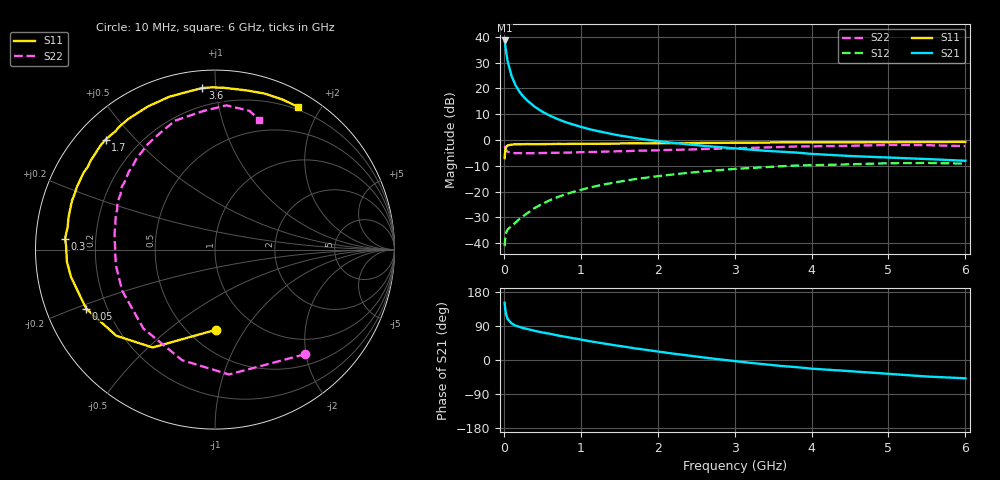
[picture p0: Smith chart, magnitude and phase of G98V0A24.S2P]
! SIEMENS Small Signal Semiconductors
! BFG235
! Si NPN RF Bipolar Junction Transistor in SOT223
! VCE = 8 V  IC = 240 mA
! Common Emitter S-Parameters:  July  1994
# GHz  S  MA  R  50
!  f  S11  S21  S12  S22
! GHz  MAG  ANG  MAG  ANG  MAG  ANG  MAG  ANG
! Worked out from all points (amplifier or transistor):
!   40 points, 10 MHz to 6 GHz, reference 50 ohm
!   highest |S21| = 38.6 dB at 10 MHz (marker M1)
!   |S21| within 3 dB of that: start of sweep to 23.42 MHz
!   unconditionally stable (mu >= 1): 421.9 MHz to 1.53 GHz
!   at 200 MHz: K = 0.83, MSG = 24.8 dB, |S12| = -30.7 dB
!   at 1.5 GHz: K = 1.00, MAG = 8.5 dB, |S12| = -16.1 dB
!   at 6 GHz: K = 0.89, MSG = 0.5 dB, |S12| = -9.1 dB
!   S11 on the Smith chart (normalised r, x): 10 MHz: 0.67, -0.75; 50 MHz: 0.12, -0.21; 300 MHz: 0.09, +0.04; 1.7 GHz: 0.09, +0.41; 3.6 GHz: 0.09, +0.92; 6 GHz: 0.17, +1.72
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0.01  0.4474 -89.6  85.11 150.8  0.0088 59.2  0.7689 -49.3
0.02  0.6466 -122.5  65.85 131.4  0.0139 47.0  0.7002 -83.6
0.03  0.73 -138.9  50.78 119.8  0.0163 39.9  0.6427 -106.6
0.05  0.7894 -155.4  33.39 107.9  0.0186 33.3  0.5937 -132.2
0.1  0.817 -169.3  17.51 96.7  0.0215 38.7  0.5657 -155.9
0.15  0.8279 -175.5  11.74 90.9  0.0251 45.2  0.5571 -165.9
0.2  0.8281 -179.0  8.786 87.5  0.0293 50.1  0.5594 -171.0
0.25  0.8306 178.1  7.073 84.3  0.0335 53.8  0.5563 -174.6
0.3  0.8377 175.9  5.906 81.9  0.0379 56.6  0.5567 -177.8
0.4  0.8306 171.3  4.44 77.0  0.0482 59.5  0.5566 178.2
0.5  0.8353 167.7  3.546 72.7  0.058 61.1  0.5615 174.9
0.6  0.8375 164.7  2.961 69.1  0.0684 61.0  0.5654 171.8
0.8  0.8413 158.3  2.234 61.2  0.0889 59.9  0.5699 166.5
1.1  0.8485 149.3  1.643 50.1  0.1185 56.0  0.5865 159.7
1.4  0.8536 142.2  1.314 40.2  0.1466 51.1  0.6032 153.6
1.7  0.8639 134.8  1.102 30.8  0.1747 45.8  0.6204 148.0
2.2  0.8735 123.7  0.883 16.8  0.2159 36.4  0.6475 137.8
3.2  0.8894 102.5  0.655 -7.4  0.2876 17.1  0.705 119.3
3.6  0.9026 94.5  0.596 -15.7  0.3103 8.7  0.7335 111.0
4.5  0.9041 78.9  0.491 -29.5  0.3393 -7.6  0.7751 94.7
5.5  0.9168 65.8  0.429 -43.6  0.3604 -25.8  0.7968 76.1
6  0.9198 60.0  0.397 -48.3  0.3501 -32.8  0.7648 71.2
